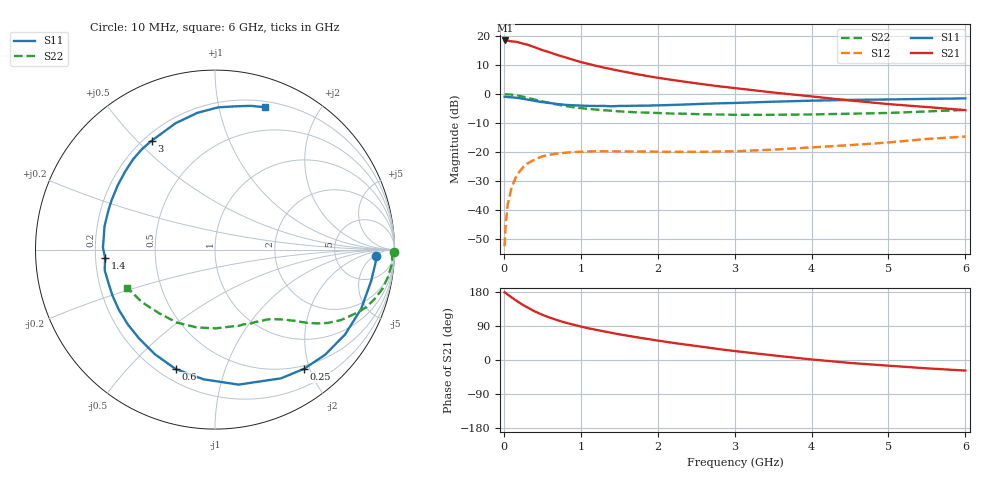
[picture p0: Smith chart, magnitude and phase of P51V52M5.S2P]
! SIEMENS Small Signal Semiconductors
! BFP183
! Si NPN RF Bipolar Junction Transistor in SOT143
! VCE = 1.5 V  IC = 2.5 mA
! Common Emitter S-Parameters:  March  1996
# GHz  S  MA  R  50
!  f  S11  S21  S12  S22
! GHz  MAG  ANG  MAG  ANG  MAG  ANG  MAG  ANG
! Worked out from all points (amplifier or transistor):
!   36 points, 10 MHz to 6 GHz, reference 50 ohm
!   highest |S21| = 18.5 dB at 20 MHz (marker M1)
!   |S21| within 3 dB of that: start of sweep to 469 MHz
!   unconditionally stable (mu >= 1): 1.927 GHz to end of sweep
!   at 250 MHz: K = 0.14, MSG = 21.3 dB, |S12| = -25.2 dB
!   at 1.4 GHz: K = 0.75, MSG = 14.1 dB, |S12| = -19.7 dB
!   at 6 GHz: K = 1.01, MAG = 4.1 dB, |S12| = -14.6 dB
!   S11 on the Smith chart (normalised r, x): 10 MHz: 16, -6; 250 MHz: 0.45, -1.91; 600 MHz: 0.26, -0.69; 1.4 GHz: 0.24, -0.04; 3 GHz: 0.23, +0.55; 6 GHz: 0.25, +1.38
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0.01  0.8984 -2.3  8.264 178.8  0.0024 89.1  0.9972 -0.9
0.02  0.8975 -4.7  8.367 177.6  0.0049 87.5  0.9883 -1.8
0.05  0.8873 -11.4  8.291 172.7  0.0125 86.4  0.9894 -4.5
0.15  0.8654 -33.1  7.973 158.3  0.0355 71.7  0.9577 -13.3
0.2  0.8484 -43.6  7.707 151.5  0.0456 66.3  0.931 -17.1
0.25  0.829 -53.3  7.368 145.1  0.0547 61.0  0.902 -20.8
0.3  0.8059 -62.9  7.121 139.6  0.0628 56.3  0.8687 -23.8
0.4  0.7636 -80.1  6.413 128.4  0.0747 48.0  0.8044 -29.2
0.5  0.7254 -95.1  5.716 119.3  0.0843 41.3  0.7484 -33.1
0.6  0.7004 -108.3  5.204 111.6  0.0906 36.1  0.698 -36.1
0.7  0.6722 -120.0  4.673 104.8  0.0944 31.6  0.6549 -38.5
0.8  0.6515 -130.3  4.28 98.7  0.0976 28.1  0.6214 -40.3
0.9  0.6403 -139.2  3.891 93.5  0.1001 25.0  0.5933 -41.9
1.1  0.6262 -155.6  3.302 83.6  0.1025 20.4  0.5534 -44.8
1.4  0.614 -175.6  2.679 71.7  0.1033 15.9  0.5151 -48.9
1.8  0.6297 163.6  2.116 57.6  0.1023 13.8  0.4812 -54.5
2.2  0.6495 146.6  1.741 45.2  0.1009 13.6  0.4608 -61.2
3  0.7016 120.2  1.268 23.7  0.1033 17.1  0.4382 -77.6
3.5  0.7374 107.4  1.063 12.2  0.1103 19.9  0.4387 -89.4
4.5  0.7928 88.7  0.775 -7.8  0.1318 22.2  0.4586 -117.5
5.5  0.8254 76.0  0.597 -22.0  0.1685 20.8  0.5015 -144.2
6  0.8413 70.5  0.528 -27.9  0.1853 17.4  0.5332 -156.6
